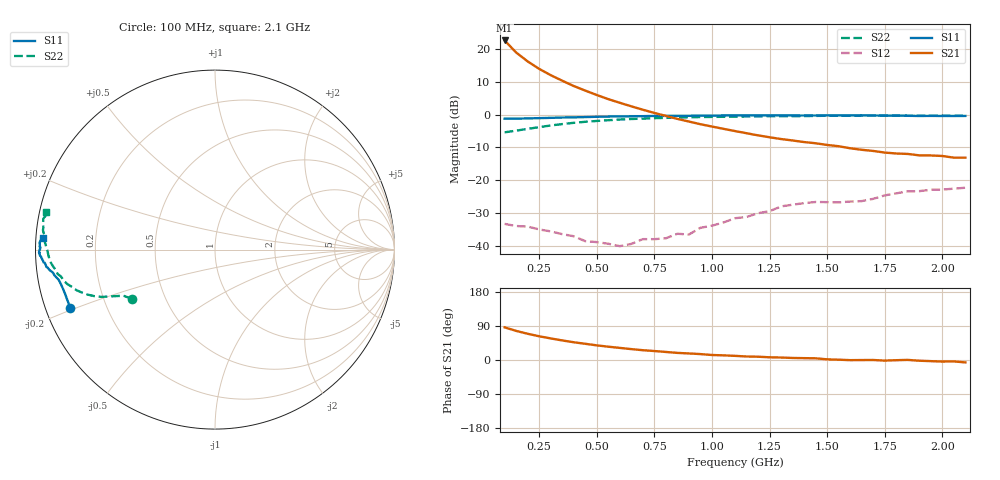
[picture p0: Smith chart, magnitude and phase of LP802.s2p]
! Tue Jun  4 13:22:41 1996
# MHZ  S  MA  R  50.0000
!  POLYFET RF DEVICES
!  LP802 - L88014
!  S PARAMETERS
!  VDS=28V, IDQ=200mA
! FREQ  S11MAG  S11ANG  S21MAG  S21ANG  S12MAG  S12ANG  S22MAG  S22ANG
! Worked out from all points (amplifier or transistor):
!   41 points, 100 MHz to 2.1 GHz, reference 50 ohm
!   highest |S21| = 22.7 dB at 100 MHz (marker M1)
!   |S21| within 3 dB of that: start of sweep to 140.8 MHz
!   unconditionally stable (mu >= 1): nowhere
!   at 400 MHz: K = 0.32, MSG = 23.0 dB, |S12| = -37.2 dB
!   at 1.1 GHz: K = -0.03, MSG = 13.3 dB, |S12| = -31.6 dB
!   at 2.1 GHz: K = -0.54, MSG = 4.6 dB, |S12| = -22.3 dB
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100  0.8696 -157.9  13.67 86.2  0.02142 4.4  0.5384 -149.4
150  0.8713 -164.0  8.95 76.8  0.01988 -2.4  0.5709 -153.2
200  0.879 -167.2  6.538 69.2  0.01949 -5.6  0.6081 -154.8
250  0.8867 -169.1  5.027 62.6  0.01764 -9.0  0.6455 -156.1
300  0.896 -169.9  4.028 57.0  0.01645 -8.6  0.6852 -157.4
350  0.9067 -171.0  3.314 51.6  0.01494 -6.0  0.7196 -158.9
400  0.912 -171.9  2.748 46.8  0.01387 -4.0  0.752 -160.5
450  0.9207 -172.5  2.34 42.8  0.01166 -0.6  0.7799 -162.1
500  0.9305 -173.1  2.002 38.6  0.01128 4.2  0.8035 -163.6
550  0.9378 -173.9  1.731 35.1  0.01065 10.8  0.8243 -165.4
600  0.9441 -174.1  1.523 31.9  0.00978 20.9  0.8448 -166.9
700  0.9509 -175.6  1.192 25.9  0.01253 36.6  0.8708 -170.1
800  0.96 -176.3  0.9602 21.2  0.01292 48.8  0.8949 -172.7
850  0.9647 -176.8  0.8637 18.7  0.01513 53.6  0.9054 -173.9
900  0.9646 -176.9  0.7869 17.3  0.01474 61.1  0.9129 -174.8
950  0.9685 -177.3  0.7158 15.6  0.01867 65.5  0.9219 -176.1
1100  0.9774 -178.5  0.5628 10.9  0.02616 66.0  0.935 -179.9
1300  0.9773 179.9  0.425 6.5  0.03965 65.5  0.9512 176.6
1450  0.9736 179.2  0.3663 4.5  0.04635 53.5  0.9592 174.5
1650  0.9788 177.8  0.2911 -0.1  0.04781 49.4  0.9681 171.8
1800  0.9718 176.2  0.2554 -0.5  0.06282 49.0  0.9722 169.9
2100  0.9589 176.0  0.2205 -6.4  0.07655 28.1  0.9629 167.6
